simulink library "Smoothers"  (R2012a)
settings: Solver=ode45  StartTime=0.0  StopTime=10.0  RelTol=1e-3

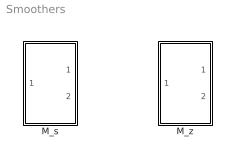
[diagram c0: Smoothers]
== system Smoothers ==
  M_s : Subsystem  mask{T=1, Q0=0}
      mask prompts: T "T_i"; Q0 "Initial Condition"
  M_z : Subsystem  mask{N=100, Ts=1, Q0=0}
      mask prompts: N "N_i"; Ts "Sampling period (Ts)"; Q0 "Initial position"

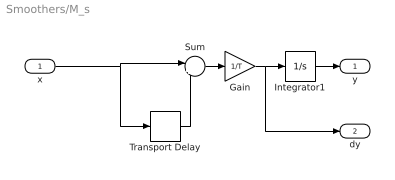
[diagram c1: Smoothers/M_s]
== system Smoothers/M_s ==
  x : Inport
  Gain : Gain  Gain=1/T
  Integrator1 : Integrator  InitialCondition=Q0
  Sum : Sum  Inputs=|+-
  Transport Delay : TransportDelay  DelayTime=T  InitialOutput=Q0  BufferSize=10000
  y : Outport
  dy : Outport  Port=2
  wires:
  Integrator1/1 -> y/1
  Gain/1 -> Integrator1/1, dy/1
  x/1 -> Transport Delay/1, Sum/1
  Transport Delay/1 -> Sum/2
  Sum/1 -> Gain/1

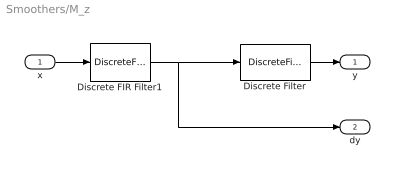
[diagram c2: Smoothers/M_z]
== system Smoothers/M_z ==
  x : Inport
  Discrete FIR Filter1 : DiscreteFir  Coefficients=1/N/Ts*[1 zeros(1,N-1) -1]  InitialStates=Q0  SampleTime=Ts
  Discrete Filter : DiscreteFilter  Numerator=[0 Ts]  Denominator=[1 -1]  InitialStates=Q0  SampleTime=Ts
  y : Outport
  dy : Outport  Port=2
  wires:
  Discrete Filter/1 -> y/1
  x/1 -> Discrete FIR Filter1/1
  Discrete FIR Filter1/1 -> dy/1, Discrete Filter/1
